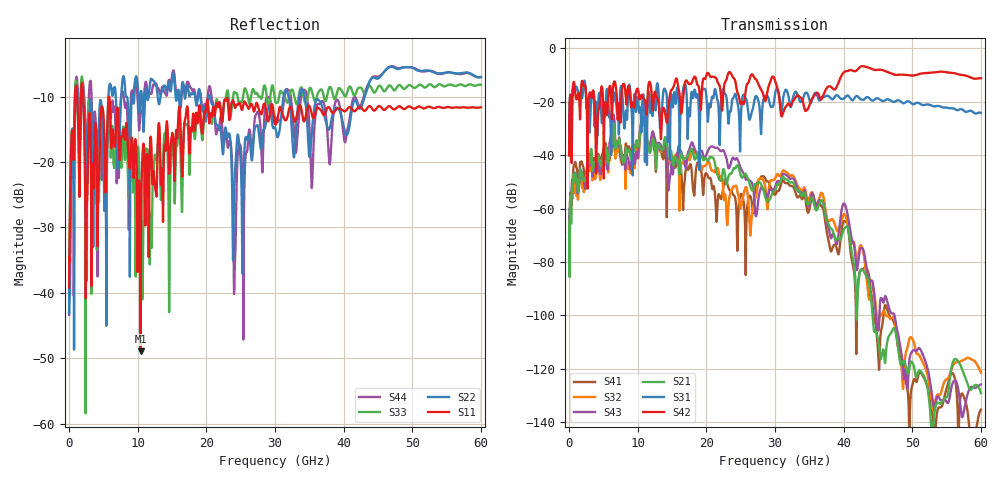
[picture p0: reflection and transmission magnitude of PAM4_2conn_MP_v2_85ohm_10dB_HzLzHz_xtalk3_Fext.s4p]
! Info: Touchstone file created by Circ.  Input file=FAB50GbE_2conn_Midplane_Examax_Topo2_v2_85ohm_10dB_HzLzHz.circ
# Hz S RI R 50
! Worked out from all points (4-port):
!   6000 points, 10 MHz to 60 GHz, reference 50 ohm
!   strongest paths, dB at 10 MHz, 15.01 GHz, 30.01 GHz, 45.01 GHz, 60 GHz:
!     S42: -40.1, -15.4, -12.0, -8.0, -11.2
!     S31: -39.6, -18.4, -17.1, -18.7, -24.1
!     S21: -64.6, -41.3, -53.2, -109.0, -129.0
!     S43: -78.5, -42.3, -52.0, -105.4, -125.8
!     S32: -69.2, -42.6, -48.7, -104.1, -121.4
!     S41: -68.5, -41.6, -54.8, -113.0, -135.3
!   lowest |S11| = -49.0 dB at 10.43 GHz (marker M1), VSWR 1.01, Z = 49.6 - j0.0155 ohm
!   |S11| at or under -10 dB: start of sweep to 877.2 MHz; 1.173 GHz to 1.728 GHz (555 MHz wide, 38.3 % of centre); 2.063 GHz to end of sweep
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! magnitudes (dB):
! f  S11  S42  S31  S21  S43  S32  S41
! 10 MHz  -39.2  -40.1  -39.6  -64.6  -78.5  -69.2  -68.5
! 1.11 GHz  -9.0  -19.1  -14.5  -49.2  -50.7  -54.0  -44.8
! 10.43 GHz  -49.0  -17.9  -23.3  -30.1  -29.4  -30.5  -28.7
! 20.53 GHz  -13.2  -10.4  -21.4  -40.6  -37.1  -43.8  -48.5
! 24.12 GHz  -11.6  -11.5  -17.3  -44.9  -41.6  -51.6  -55.3
! 41.96 GHz  -11.9  -8.1  -17.8  -99.1  -82.9  -78.9  -94.0
! 60 GHz  -11.6  -11.2  -24.1  -129.0  -125.8  -121.4  -135.3
